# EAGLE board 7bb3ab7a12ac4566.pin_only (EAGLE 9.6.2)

Size 23 x 23 mm. Coordinates in mm from the lower left corner, seen from the top.
Outline: 0,3 0,20 arc-90 3,23 20,23 arc-90 23,20 23,3 arc-90 20,0 3,0 arc-90 0,3
Copper layers (1*16): Top 0.035mm / dielectric 1.5mm / Bottom 0.035mm
Design rules "default *": minimum track width 10mil, minimum drill 19mil, track to track 8mil, track to pad 8mil, pad to pad 8mil, via to via 8mil, smd to smd 8mil, copper to edge 40mil, drill to drill 8mil, minimum pad ring 10mil, minimum via ring 8mil, stop-mask expansion 4mil, vias tented up to drill 24mil, thermal gap 10mil

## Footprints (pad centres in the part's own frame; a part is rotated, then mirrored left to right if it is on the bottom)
0805 = smd 1.3 x 1.5: 1 -0.95,0; 2 0.95,0
1X05_ROUND_76 = drill 1 pad 1.93: 1 -5.08,0; 2 -2.54,0; 3 0,0; 4 2.54,0; 5 5.08,0
VCNL4000 = smd 0.35 x 0.805: 1 -1.5,-1.772; 2 -0.75,-1.772; 3 0,-1.772; 4 0.75,-1.772; 5 1.5,-1.772; 7 1.5,1.772; 8 0.75,1.772; 9 0,1.772; 10 -0.75,1.772; 11 -1.5,1.772 | smd 0.805 x 0.4: 6 1.772,-0.715; 12 -1.772,-0.2
SOT23-5 = smd 0.55 x 1.2: 1 -0.95,-1.3; 2 0,-1.3; 3 0.95,-1.3; 4 0.95,1.3; 5 -0.95,1.3
MOUNTINGHOLE_2.0_PLATED = drill 2 pad 3: P$1 0,0
FIDUCIAL_1MM = smd 1 x 1: 1 0,0

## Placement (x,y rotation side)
C1  10uF  [0805]  16.43,10.49 0 top
C2  10uF  [0805]  5.08,16.51 180 top
C3  0.1uF  [0805]  3.06,5.08 180 top
C4  10uF  [0805]  16.43,15.55 0 top
C6  10uF  [0805]  16.43,13.51 0 top
JP1  [1X05_ROUND_76]  11.5,2.54 0 top
R1  10K  [0805]  3.04,10.16 180 top
R2  10K  [0805]  3.04,7.62 180 top
U1  VCNL4000-GS08  [VCNL4000]  11.43,12.7 270 top
U2  AP7311-33  [SOT23-5]  5.08,12.97 90 top
U$5  MOUNTINGHOLE2.0  [MOUNTINGHOLE_2.0_PLATED]  3,20 0 top
U$6  MOUNTINGHOLE2.0  [MOUNTINGHOLE_2.0_PLATED]  20,20 0 top
U$7  FIDUCIAL  [FIDUCIAL_1MM]  20.32,16.51 0 top
U$8  FIDUCIAL  [FIDUCIAL_1MM]  2.29,2.03 0 top
U$13  [ADAFRUIT200MIL]  20.23,2.6 270 top

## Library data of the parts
C1-C4 C6 JP1 R1 R2 U1 U2 U$5 U$6 = microbuilder
U$7 U$8 U$13 = adafruit

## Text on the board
tPlace: VCNL4000 | Proximity | Sensor | 3.3V | SCL | SDA | GND | Vin
bPlace: VCNL4000 | Proximity | Sensor | ~1-200mm range | VIN: 3.3-5.0V | Logic: 3.3-5.0V | VOUT: 3.3V (100mA) | Adafruit Industries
